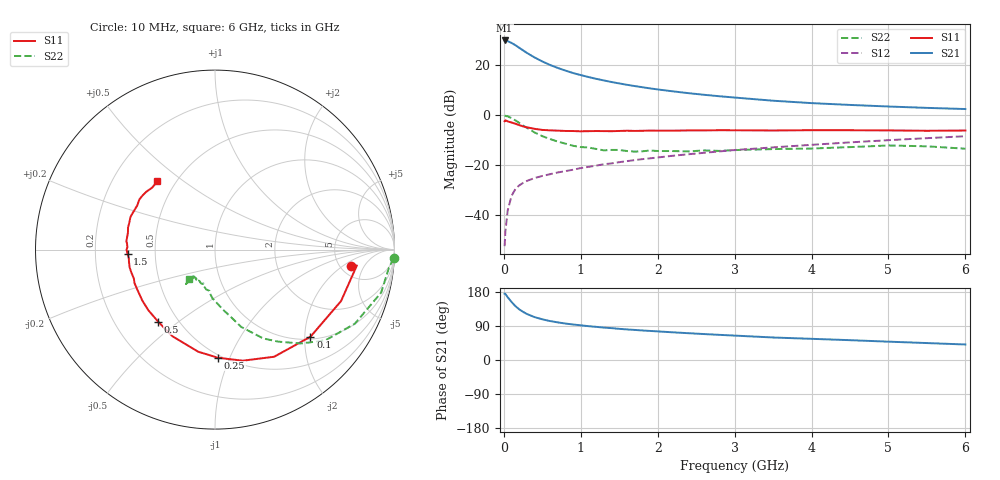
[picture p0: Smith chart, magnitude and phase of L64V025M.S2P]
!  INFINEON TECHNOLOGIES Small Signal Semiconductors
! BFR380L3 , Si-NPN RF-Transistor in TSLP-3-1
!  Vce=4 V,  Ic=25 mA
! Common Emitter S-Parameters:  07. March 2005
#  GHz  S  MA  R  50
! f  S11  S21  S12  S22
! GHz  Mag  Ang  Mag  Ang  Mag  Ang  Mag  Ang
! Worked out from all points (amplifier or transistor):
!   36 points, 10 MHz to 6 GHz, reference 50 ohm
!   highest |S21| = 30.0 dB at 10 MHz (marker M1)
!   |S21| within 3 dB of that: start of sweep to 202.9 MHz
!   unconditionally stable (mu >= 1): 1.988 GHz to 4.75 GHz
!   at 250 MHz: K = 0.35, MSG = 26.6 dB, |S12| = -27.1 dB
!   at 1.4 GHz: K = 0.94, MSG = 16.3 dB, |S12| = -19.2 dB
!   at 6 GHz: K = 0.97, MSG = 5.4 dB, |S12| = -8.3 dB
!   S11 on the Smith chart (normalised r, x): 10 MHz: 6.25, -2.70; 100 MHz: 1.06, -2.13; 250 MHz: 0.48, -0.90; 500 MHz: 0.39, -0.42; 1.5 GHz: 0.34, -0.02; 6 GHz: 0.40, +0.40
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0.01  0.7631 -6.8  31.69 175.1  0.0024 78.2  0.9967 -2.8
0.02  0.7953 -6.4  31.68 174.3  0.0047 88.1  0.9742 -6.0
0.05  0.7586 -22.2  30.68 165.7  0.0125 80.8  0.9562 -14.5
0.1  0.7201 -42.4  28.28 153.2  0.0243 71.8  0.882 -27.9
0.15  0.6819 -61.1  25.51 142.3  0.0335 64.1  0.7957 -39.5
0.2  0.638 -76.0  22.59 133.7  0.0396 59.8  0.7083 -47.6
0.25  0.6025 -88.5  20.07 127.1  0.0444 55.5  0.6232 -55.4
0.3  0.5765 -99.4  17.82 121.4  0.0487 53.9  0.5635 -61.5
0.4  0.5377 -116.3  14.46 113.1  0.0556 52.0  0.4548 -71.3
0.5  0.5113 -128.4  12.04 107.4  0.0612 52.2  0.3838 -76.9
0.6  0.5019 -137.8  10.24 102.8  0.0663 52.2  0.3363 -82.6
0.7  0.4947 -144.8  8.928 99.3  0.0719 53.8  0.2988 -87.8
0.9  0.4858 -157.5  7.058 93.7  0.0815 55.9  0.246 -96.6
1.1  0.4832 -164.6  5.863 89.3  0.093 57.6  0.2274 -102.4
1.5  0.4875 -177.1  4.367 82.2  0.1155 60.4  0.2034 -112.6
1.8  0.4913 176.1  3.667 77.9  0.1329 61.6  0.1909 -118.2
2.2  0.4942 169.0  3.029 73.0  0.1555 62.3  0.1929 -122.3
2.8  0.5046 159.2  2.42 66.4  0.1896 63.3  0.1944 -129.5
3.5  0.4982 150.3  1.967 59.4  0.2287 61.9  0.2113 -129.7
4.5  0.5042 143.8  1.62 52.3  0.2881 61.1  0.2314 -130.1
5.5  0.4917 135.5  1.414 44.7  0.3499 57.9  0.2401 -130.1
6  0.4976 130.1  1.34 40.9  0.3825 56.0  0.215 -131.5
